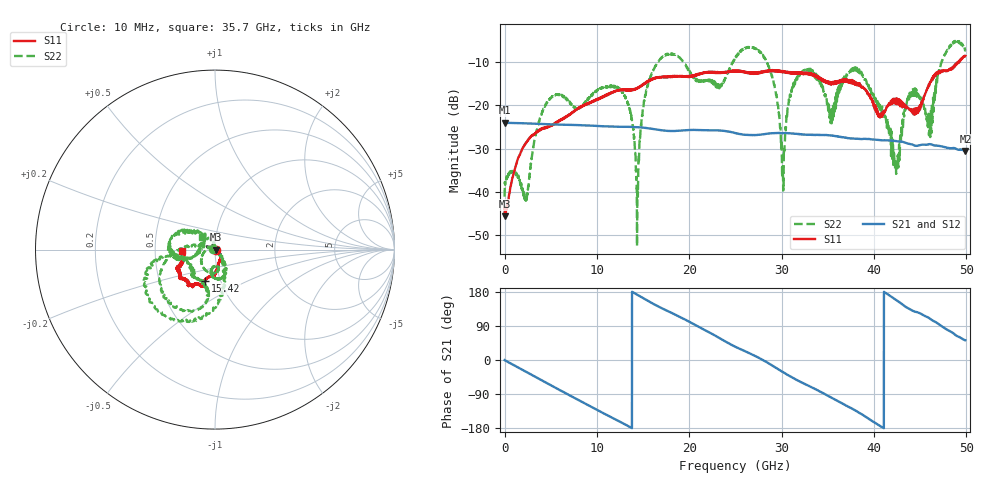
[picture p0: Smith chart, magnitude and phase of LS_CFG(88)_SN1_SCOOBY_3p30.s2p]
!Keysight Technologies,N5245B,MY58422026,A.13.80.08
!Date: Thursday, March 19, 2020 23:54:40
!Correction: S11(Full 2 Port(1,2))
!S21(Full 2 Port(1,2))
!S12(Full 2 Port(1,2))
!S22(Full 2 Port(1,2))
!S2P File: Measurements: S11, S21, S12, S22:
# Hz S DB R 50.0
!freq dBS11 angS11 dBS21 angS21 dBS12 angS12 dBS22 angS22
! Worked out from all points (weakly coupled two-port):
!   4991 points, 10 MHz to 49.91 GHz, reference 50 ohm
!   highest |S21| = -24.03 dB at 10 MHz (marker M1); lowest = -30.6 dB at 49.91 GHz (marker M2)
!   lowest |S11| = -45.6 dB at 30 MHz (marker M3), VSWR 1.01, Z = 50.5 - j0.0252 ohm
!   |S11| at or under -10 dB: start of sweep to 49.13 GHz; 49.16429 GHz to 49.22625 GHz (61.97 MHz wide, 0.126 % of centre)
!   |S22| runs from -52.5 to -5.1 dB; largest |S21 - S12| = 0.00067
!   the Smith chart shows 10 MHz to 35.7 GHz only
!   S11 on the Smith chart (normalised r, x): 10 MHz: 1.01, -0.01; 15.42 GHz: 0.84, -0.30; 35.7 GHz: 0.69, -0.02
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1e7  -43.87 -27.3  -24.03 -0.3  -24.03 -0.3  -41.09 174.0
3e7  -45.64 -2.7  -24.04 -0.5  -24.04 -0.5  -38.33 -173.3
2.34e9  -28.59 -39.8  -24.20 -31.5  -24.19 -31.4  -41.69 60.7
4.91e9  -24.73 -57.0  -24.42 -65.4  -24.41 -65.4  -18.48 -124.0
8.33e9  -20.42 -80.3  -24.63 -110.1  -24.63 -110.0  -20.29 -95.1
1.267e10  -16.54 -91.6  -24.98 -165.0  -24.98 -165.0  -16.68 -67.8
1.436e10  -16.16 -103.3  -25.06 172.4  -25.06 172.5  -48.40 -96.0
1.542e10  -14.76 -107.8  -25.28 157.6  -25.28 157.7  -16.24 172.6
1.665e10  -13.64 -107.7  -25.68 141.3  -25.68 141.4  -9.94 -158.9
2.496e10  -12.18 -127.3  -26.40 35.3  -26.39 35.5  -9.29 -167.5
2.838e10  -12.03 -139.2  -26.61 -5.5  -26.61 -5.2  -9.78 -89.1
3.015e10  -12.24 -144.3  -26.46 -31.8  -26.46 -31.6  -35.67 42.3
3.116e10  -12.52 -147.1  -26.54 -46.1  -26.55 -45.8  -15.81 142.9
3.328e10  -12.88 -156.1  -26.84 -72.5  -26.83 -72.1  -12.11 -174.2
3.57e10  -14.63 -176.2  -27.12 -103.3  -27.06 -102.8  -19.50 141.3
3.816e10  -15.38 176.8  -27.76 -135.5  -27.71 -135.7  -11.39 -175.4
4.16e10  -19.70 106.2  -28.15 171.8  -28.16 171.6  -24.95 69.7
4.245e10  -18.67 105.6  -28.30 157.7  -28.32 157.5  -35.31 -176.2
4.39e10  -20.96 77.1  -28.93 134.0  -28.94 134.0  -17.41 -31.8
4.601e10  -15.39 5.7  -28.98 110.0  -29.00 110.1  -23.36 114.2
4.771e10  -12.05 5.8  -29.70 82.9  -29.71 83.1  -8.14 -79.6
4.991e10  -8.63 -14.1  -30.56 52.1  -30.57 52.1  -7.32 -15.0
